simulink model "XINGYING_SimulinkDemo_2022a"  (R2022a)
settings: Solver=VariableStepAuto  StartTime=0.0  StopTime=1000.0  RelTol=1e-3
libraries: sldrtlib x1

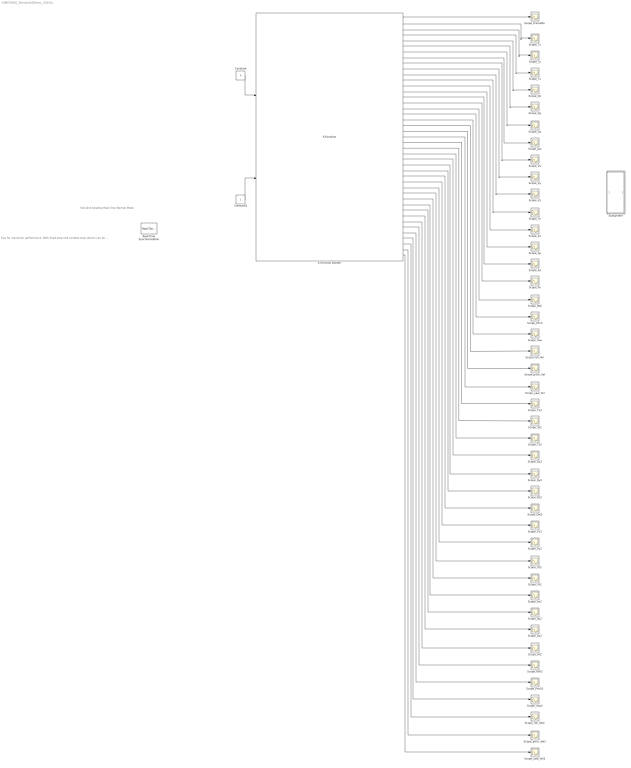
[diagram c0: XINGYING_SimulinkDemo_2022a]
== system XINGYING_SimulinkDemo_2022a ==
  note: Simulink Desktop Real-Time Normal Mode
  note: Tips for maximum performance: Both fixed-step and variable-step solvers can be used in Normal mode. All I/O blocks perform real-time synchronizaton. Use the Real-Time Synchronization block only if no I/O block is used. Use a single block that reads or writes all channels of given type, rather than multiple blocks for one channel each.
  Constant : Constant  Value=0  OutDataTypeStr=int32
  Constant2 : Constant  OutDataTypeStr=int32
  Real-Time Synchronization : sldrtlib/Real-Time Synchronization  Commented=on  SampleTime=0.1  MaxMissedTicks=10  ShowMissedTicks=off  YieldWhenWaiting=off
  S-Function Builder : S-Function  InitFcn=try, set_param(gcb,'FunctionName','Get_Data_From_XINGYING_API'), end  FunctionName=Get_Data_From_XINGYING_API  SFunctionModules=Get_Data_From_XINGYING_API_wrapper  SFunctionDeploymentMode=off  EnableBusSupport=off  mask(S-Function Builder){}
      mask help: Simulink:masks:SFunctionBuilder_MD
      mask init:
      | val = [[.9  0.75 0.75 1 1 .9 .9 1]',[1 1 0.75 0.75 .9 .9 1 .9]'];try , sys = get_param(gcb,'SfunBuilderFcnName');if isempty(sys), sys = get_param(gcb,'FunctionName'); end,catch, sys = get_param(gcb,'FunctionName'); end
  Scope_Ar : Scope
  Scope_Ar2 : Scope
  Scope_Ax : Scope
  Scope_Ax2 : Scope
  Scope_Ay : Scope
  Scope_Ay2 : Scope
  Scope_Az : Scope
  Scope_Az2 : Scope
  "Scope_FrameNo " : Scope
  Scope_Pitch : Scope
  Scope_Pitch2 : Scope
  Scope_Qw : Scope
  Scope_Qw2 : Scope
  Scope_Qx : Scope
  Scope_Qx2 : Scope
  Scope_Qy : Scope
  Scope_Qy2 : Scope
  Scope_Qz : Scope
  Scope_Qz2 : Scope
  Scope_Roll : Scope
  Scope_Roll2 : Scope
  Scope_Tx : Scope
  Scope_Tx2 : Scope
  Scope_Ty : Scope
  Scope_Ty2 : Scope
  Scope_Tz : Scope
  Scope_Tz2 : Scope
  Scope_Vr : Scope
  Scope_Vr2 : Scope
  Scope_Vx : Scope
  Scope_Vx2 : Scope
  Scope_Vy : Scope
  Scope_Vy2 : Scope
  Scope_Vz : Scope
  Scope_Vz2 : Scope
  Scope_Yaw : Scope
  Scope_Yaw2 : Scope
  Scope_pitch_Vel : Scope
  Scope_pitch_Vel2 : Scope
  Scope_roll_Vel : Scope
  Scope_roll_Vel2 : Scope
  Scope_yaw_Vel : Scope
  Scope_yaw_Vel2 : Scope
  Subsystem : Subsystem
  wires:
  S-Function Builder/4 -> Scope_Tz/1
  S-Function Builder/36 -> Scope_Az2/1
  S-Function Builder/37 -> Scope_Ar2/1
  S-Function Builder/38 -> Scope_Roll2/1
  S-Function Builder/21 -> Scope_pitch_Vel/1
  S-Function Builder/39 -> Scope_Pitch2/1
  S-Function Builder/13 -> Scope_Ax/1
  S-Function Builder/32 -> Scope_Vz2/1
  S-Function Builder/40 -> Scope_Yaw2/1
  Constant/1 -> S-Function Builder/1
  S-Function Builder/31 -> Scope_Vy2/1
  S-Function Builder/33 -> Scope_Vr2/1
  S-Function Builder/41 -> Scope_roll_Vel2/1
  S-Function Builder/34 -> Scope_Ax2/1
  S-Function Builder/42 -> Scope_pitch_Vel2/1
  S-Function Builder/8 -> Scope_Qw/1
  S-Function Builder/35 -> Scope_Ay2/1
  S-Function Builder/43 -> Scope_yaw_Vel2/1
  S-Function Builder/29 -> Scope_Qw2/1
  S-Function Builder/30 -> Scope_Vx2/1
  S-Function Builder/27 -> Scope_Qy2/1
  S-Function Builder/28 -> Scope_Qz2/1
  S-Function Builder/26 -> Scope_Qx2/1
  S-Function Builder/25 -> Scope_Tz2/1
  S-Function Builder/24 -> Scope_Ty2/1
  S-Function Builder/23 -> Scope_Tx2/1
  S-Function Builder/22 -> Scope_yaw_Vel/1
  S-Function Builder/20 -> Scope_roll_Vel/1
  S-Function Builder/19 -> Scope_Yaw/1
  S-Function Builder/18 -> Scope_Pitch/1
  S-Function Builder/17 -> Scope_Roll/1
  S-Function Builder/16 -> Scope_Ar/1
  S-Function Builder/15 -> Scope_Az/1
  S-Function Builder/14 -> Scope_Ay/1
  S-Function Builder/12 -> Scope_Vr/1
  S-Function Builder/11 -> Scope_Vz/1
  S-Function Builder/10 -> Scope_Vy/1
  S-Function Builder/9 -> Scope_Vx/1
  Constant2/1 -> S-Function Builder/2
  S-Function Builder/7 -> Scope_Qz/1
  S-Function Builder/6 -> Scope_Qy/1
  S-Function Builder/5 -> Scope_Qx/1
  S-Function Builder/3 -> Scope_Ty/1
  S-Function Builder/2 -> Scope_Tx/1
  S-Function Builder/1 -> "Scope_FrameNo "/1

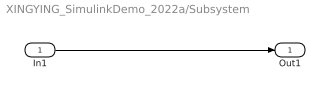
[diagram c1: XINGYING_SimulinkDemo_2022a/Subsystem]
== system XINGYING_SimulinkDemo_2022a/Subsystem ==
  In1 : Inport
  Out1 : Outport
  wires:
  In1/1 -> Out1/1
